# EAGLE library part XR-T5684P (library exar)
T1 LINE INTERFACE
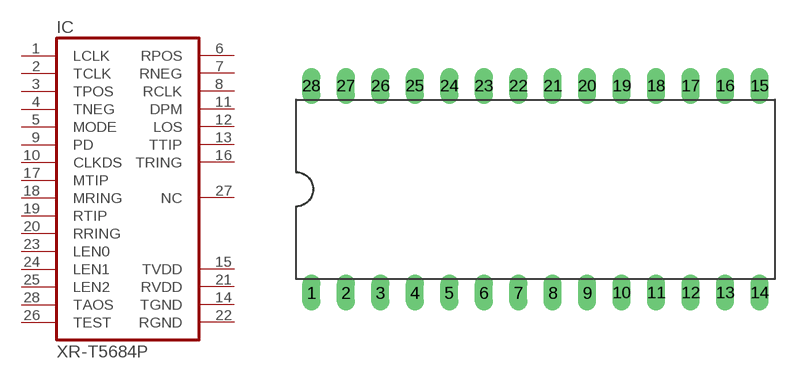
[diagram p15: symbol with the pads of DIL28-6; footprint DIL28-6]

Designator prefix IC

## XR-T5684P (OC_FARNELL: unknown; OC_NEWARK: unknown)  [DIL28-6]
1  LCLK  in
2  TCLK  in
3  TPOS  in
4  TNEG  in
5  MODE  in
6  RPOS  out
7  RNEG  out
8  RCLK  out
9  PD  in
10  CLKDS  in
11  DPM  out
12  LOS  out
13  TTIP  out
14  TGND  pwr
15  TVDD  pwr
16  TRING  out
17  MTIP  in
18  MRING  in
19  RTIP  in
20  RRING  in
21  RVDD  pwr
22  RGND  pwr
23  LEN0  in
24  LEN1  in
25  LEN2  in
26  TEST  in
27  NC  nc
28  TAOS  in

## Footprint DIL28-6 (pad centres in mm)
Dual In Line Package 0.6 inch
drill 0.813 long: 1 -16.51,-7.62; 2 -13.97,-7.62; 3 -11.43,-7.62; 4 -8.89,-7.62; 5 -6.35,-7.62; 6 -3.81,-7.62; 7 -1.27,-7.62; 8 1.27,-7.62; 9 3.81,-7.62; 10 6.35,-7.62; 11 8.89,-7.62; 12 11.43,-7.62; 13 13.97,-7.62; 14 16.51,-7.62; 15 16.51,7.62; 16 13.97,7.62; 17 11.43,7.62; 18 8.89,7.62; 19 6.35,7.62; 20 3.81,7.62; 21 1.27,7.62; 22 -1.27,7.62; 23 -3.81,7.62; 24 -6.35,7.62; 25 -8.89,7.62; 26 -11.43,7.62; 27 -13.97,7.62; 28 -16.51,7.62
